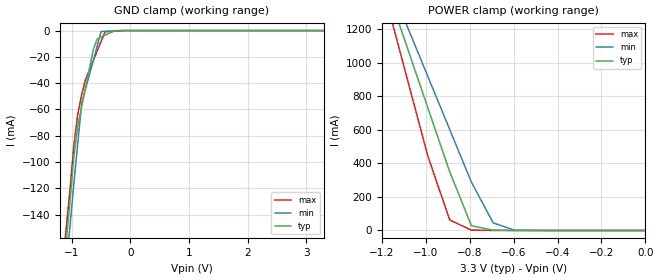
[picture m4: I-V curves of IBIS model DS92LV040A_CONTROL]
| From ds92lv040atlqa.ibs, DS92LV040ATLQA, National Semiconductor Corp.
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[Model]   DS92LV040A_CONTROL
Model_type Input
Vinh=2.0
Vinl=0.8
C_comp   3.834p   3.834p   3.834p
[Model Spec]
S_overshoot_high   3.6   3.3   3.9
S_overshoot_low   -0.3   -0.3   -0.3
[Temperature Range] 25   85   -40
[Voltage Range]   3.3   3.00   3.60
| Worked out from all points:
|   GND clamp passes 1 mA (typ) near -0.31 V on its own axis
|   POWER clamp passes 1 mA (typ) near -0.65 V on its own axis
[GND Clamp]
-3.3V     -1.36A     -1.35A     -1.39A
-1.1V     -162mA     -179mA     -152mA
-1.03V    -129mA     -148mA     -120mA
-967mV    -96.5mA    -117mA     -87.8mA
-900mV    -72.8mA    -86.2mA    -63.9mA
-833mV    -58.1mA    -55.4mA    -48.9mA
-633mV    -14.3mA    -22.6mA    -22.7mA
-567mV    -6.25mA    -11.6mA    -15.4mA
-500mV    -4.86mA    -677uA     -8.17mA
-433mV    -3.47mA    -541uA     -919uA
-100mV    -2.96uA    -229nA     -6.79nA
3.3V      910pA      1.9nA      287pA
[POWER Clamp]
-3.267V   9.584A     8.291A     11.75A
-1.188V   1.491A     1.55A      1.416A
-1.089V   1.11A      1.233A     928.2mA
-990mV    729.5mA    917.3mA    441.9mA
-891mV    350.5mA    602.3mA    63.05mA
-792mV    28.24mA    288.1mA    1.817mA
-693mV    1.617mA    45.27mA    453.5uA
-594mV    118.9uA    1.221mA    66.77uA
0V        857.1pA    1.83nA     132.3pA
